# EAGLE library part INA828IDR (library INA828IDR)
50-uV Offset, 7-nV/Hz Noise, Low-Power, Precision Instrumentation Amplifier Source: Datasheet
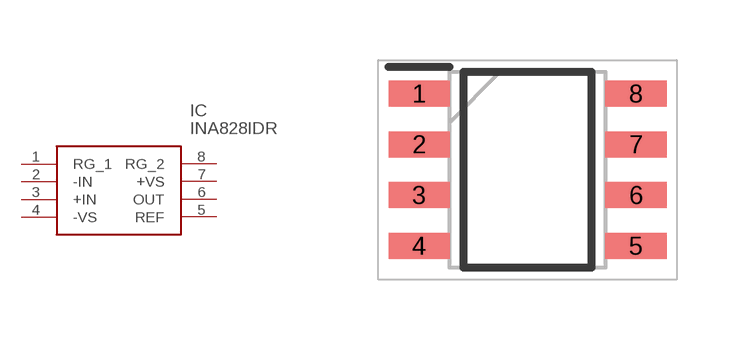
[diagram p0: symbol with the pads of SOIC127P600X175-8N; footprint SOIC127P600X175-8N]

Designator prefix IC

## INA828IDR (Arrow_Part_Number: INA828IDR; Arrow_Price-Stock: https://www.arrow.com/en/products/ina828idr/texas-instruments?region=nac; Description: 50-uV Offset, 7-nV/Hz Noise, Low-Power, Precision Instrumentation Amplifier; Height: 1.75mm; Manufacturer_Name: Texas Instruments; Manufacturer_Part_Number: INA828IDR; Mouser_Part_Number: 595-INA828IDR; Mouser_Price-Stock: https://www.mouser.co.uk/ProductDetail/Texas-Instruments/INA828IDR?qs=YCa%2FAAYMW01L8%252BXCfEPVuA%3D%3D)  [SOIC127P600X175-8N]
1  RG_1
2  -IN
3  +IN
4  -VS
5  REF
6  OUT
7  +VS
8  RG_2

## Footprint SOIC127P600X175-8N (pad centres in mm)
8-Pin SOIC-ren5
smd 1.528 x 0.65: 1 -2.711,1.905; 2 -2.711,0.635; 3 -2.711,-0.635; 4 -2.711,-1.905; 5 2.711,-1.905; 6 2.711,-0.635; 7 2.711,0.635; 8 2.711,1.905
